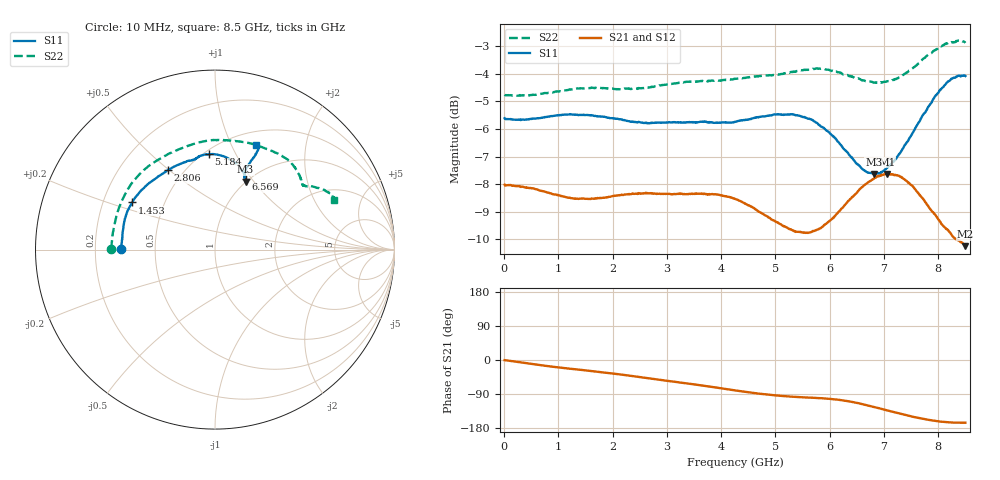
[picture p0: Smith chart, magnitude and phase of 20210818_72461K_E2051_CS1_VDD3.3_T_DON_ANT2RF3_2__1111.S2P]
!Agilent Technologies,E5071C,MY46417908,A.11.23
!Date: Wed Aug 18 14:31:15 2021
!Data & Calibration Information:
!Freq	S11:SOLT2(ON)	S21:SOLT2(ON)	S12:SOLT2(ON)	S22:SOLT2(ON)
!PortZ  Port1:50+j0  Port2:50+j0
!Above PortZ is port z conversion or system Z0 setting when saving the data.
!When reading, reference impedance value at option line is always used.
# Hz S dB R 50
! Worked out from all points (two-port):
!   1601 points, 10 MHz to 8.5 GHz, reference 50 ohm
!   highest |S21| = -7.63 dB at 7.057 GHz (marker M1); lowest = -10.2 dB at 8.5 GHz (marker M2)
!   |S21| within 3 dB of the highest: start of sweep to end of sweep
!   lowest |S11| = -7.6 dB at 6.813 GHz (marker M3), VSWR 2.42, Z = 49.7 + j45.6 ohm
!   |S11| at or under -10 dB: nowhere
!   |S22| runs from -4.8 to -2.8 dB; largest |S21 - S12| = 0.0024
!   S11 on the Smith chart (normalised r, x): 10 MHz: 0.31, +0.00; 1.453 GHz: 0.33, +0.24; 2.806 GHz: 0.41, +0.49; 5.184 GHz: 0.53, +0.79; 6.569 GHz: 0.97, +0.93; 8.5 GHz: 0.66, +1.25
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1e7  -5.61 179.7  -8.02 -0.4  -8.02 -0.3  -4.76 179.6
7.741e8  -5.57 164.9  -8.28 -15.6  -8.28 -15.6  -4.70 158.6
1.426769e9  -5.49 151.0  -8.52 -26.2  -8.52 -26.2  -4.53 139.3
1.4533e9  -5.49 150.4  -8.52 -26.6  -8.53 -26.6  -4.53 138.5
2.137806e9  -5.65 135.2  -8.39 -38.0  -8.40 -38.0  -4.57 119.0
2.806394e9  -5.77 120.8  -8.35 -51.1  -8.34 -51.2  -4.46 102.8
2.843538e9  -5.77 120.2  -8.34 -51.8  -8.34 -51.9  -4.44 102.0
3.586412e9  -5.75 108.0  -8.34 -66.1  -8.33 -66.1  -4.28 88.0
4.255e9  -5.75 102.3  -8.53 -80.2  -8.52 -80.2  -4.19 77.3
4.780319e9  -5.55 98.9  -9.09 -90.2  -9.08 -90.1  -4.07 69.1
5.183594e9  -5.48 93.6  -9.54 -95.6  -9.55 -95.5  -3.98 61.6
5.671769e9  -5.67 84.0  -9.72 -99.5  -9.74 -99.5  -3.84 52.6
6.149331e9  -6.46 72.7  -9.03 -104.7  -9.06 -104.9  -3.95 44.5
6.568525e9  -7.38 66.4  -8.15 -115.2  -8.15 -115.3  -4.21 38.8
6.812612e9  -7.62 65.8  -7.81 -123.6  -7.81 -123.7  -4.33 37.0
7.0567e9  -7.40 66.9  -7.63 -132.9  -7.63 -132.9  -4.27 35.6
7.088538e9  -7.35 67.3  -7.63 -134.0  -7.64 -134.1  -4.27 35.6
7.337931e9  -6.73 68.8  -7.76 -143.2  -7.76 -143.2  -4.06 34.4
7.571406e9  -5.99 68.5  -8.18 -151.1  -8.18 -151.1  -3.74 32.6
8.048969e9  -4.57 66.7  -9.41 -162.7  -9.37 -162.8  -3.01 26.9
8.351425e9  -4.09 67.5  -10.02 -165.2  -9.98 -165.2  -2.81 23.7
8.5e9  -4.09 68.4  -10.24 -165.5  -10.18 -165.5  -2.88 22.6
